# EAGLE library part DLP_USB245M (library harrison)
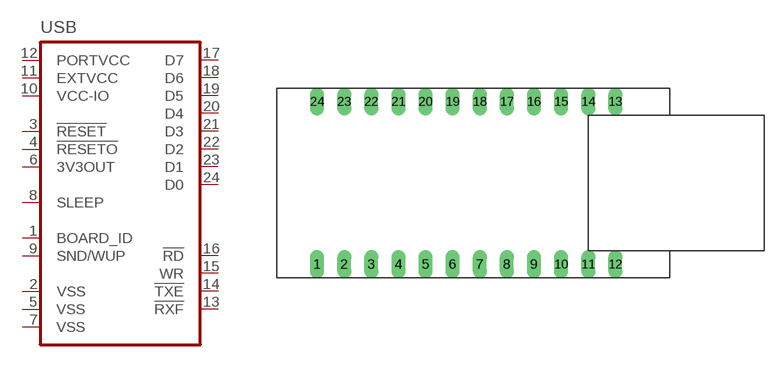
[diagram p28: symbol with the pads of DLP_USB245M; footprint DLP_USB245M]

Designator prefix USB

## DLP_USB245M  [DLP_USB245M]
1  BOARD_ID  out
2  VSS  pwr
3  !RESET!  in
4  !RESETO!  out
5  VSS  pwr
6  3V3OUT  pwr
7  VSS  pwr
8  SLEEP  out
9  SND/WUP  in
10  VCC-IO  pwr
11  EXTVCC  pwr
12  PORTVCC  pwr
13  !RXF  out
14  !TXE!  out
15  WR  in
16  !RD!  in
17  D7
18  D6
19  D5
20  D4
21  D3
22  D2
23  D1
24  D0

## Footprint DLP_USB245M (pad centres in mm)
drill 0.813 long: 1 -13.97,-7.62; 2 -11.43,-7.62; 3 -8.89,-7.62; 4 -6.35,-7.62; 5 -3.81,-7.62; 6 -1.27,-7.62; 7 1.27,-7.62; 8 3.81,-7.62; 9 6.35,-7.62; 10 8.89,-7.62; 11 11.43,-7.62; 12 13.97,-7.62; 13 13.97,7.62; 14 11.43,7.62; 15 8.89,7.62; 16 6.35,7.62; 17 3.81,7.62; 18 1.27,7.62; 19 -1.27,7.62; 20 -3.81,7.62; 21 -6.35,7.62; 22 -8.89,7.62; 23 -11.43,7.62; 24 -13.97,7.62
